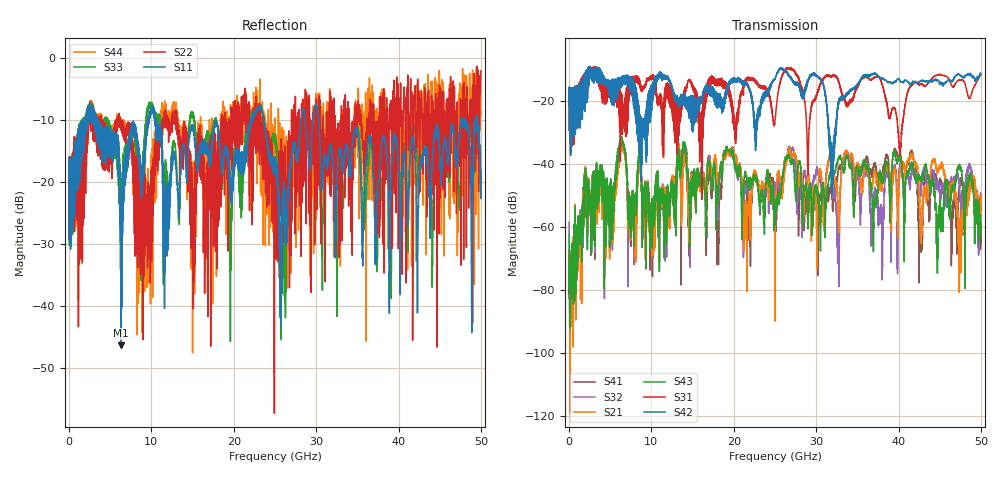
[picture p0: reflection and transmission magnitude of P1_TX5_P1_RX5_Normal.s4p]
!Keysight Technologies,N5225B,MY57041031,A.13.20.10
!Date: Friday, May 31, 2019 11:20:57
!Correction: S11(Full 4 Port(1,2,3,4))
!S12(Full 4 Port(1,2,3,4))
!S13(Full 4 Port(1,2,3,4))
!S14(Full 4 Port(1,2,3,4))
!S21(Full 4 Port(1,2,3,4))
!S22(Full 4 Port(1,2,3,4))
!S23(Full 4 Port(1,2,3,4))
!S24(Full 4 Port(1,2,3,4))
!S31(Full 4 Port(1,2,3,4))
!S32(Full 4 Port(1,2,3,4))
!S33(Full 4 Port(1,2,3,4))
!S34(Full 4 Port(1,2,3,4))
!S41(Full 4 Port(1,2,3,4))
!S42(Full 4 Port(1,2,3,4))
!S43(Full 4 Port(1,2,3,4))
!S44(Full 4 Port(1,2,3,4))
!S4P File: Measurements: <S11,S12,S13,S14>,
!<S21,S22,S23,S24>,
!<S31,S32,S33,S34>,
!<S41,S42,S43,S44>:
# Hz S  dB  R 50.0
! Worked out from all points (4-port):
!   5000 points, 10 MHz to 50 GHz, reference 50 ohm
!   strongest paths, dB at 10 MHz, 12.51 GHz, 25.01 GHz, 37.51 GHz, 50 GHz:
!     S42: -19.6, -15.7, -13.1, -12.3, -11.7
!     S31: -19.4, -23.0, -26.1, -12.3, -11.7
!     S43: -62.2, -46.0, -55.5, -47.7, -59.8
!     S21: -67.1, -44.1, -65.1, -47.2, -53.4
!     S32: -58.5, -45.8, -46.7, -55.1, -52.8
!     S41: -68.8, -44.1, -50.9, -43.8, -59.7
!   lowest |S11| = -46.4 dB at 6.34 GHz (marker M1), VSWR 1.01, Z = 49.6 - j0.26 ohm
!   |S11| at or under -10 dB: 3.502 GHz to 9.556 GHz (6.054 GHz wide, 92.7 % of centre); 10.5 GHz to 22.11 GHz (11.6 GHz wide, 71.2 % of centre); 30.29 GHz to 47.6 GHz (17.31 GHz wide, 44.4 % of centre)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
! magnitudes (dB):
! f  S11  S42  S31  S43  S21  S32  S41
! 10 MHz  -19.8  -19.6  -19.4  -62.2  -67.1  -58.5  -68.8
! 6.34 GHz  -46.4  -15.7  -20.3  -31.2  -32.9  -31.9  -32.1
! 10 GHz  -8.0  -15.8  -12.9  -54.7  -53.7  -54.6  -53.1
! 25.8 GHz  -37.9  -9.6  -12.6  -46.6  -47.7  -47.3  -45.0
! 29.88 GHz  -7.8  -11.6  -19.1  -47.8  -48.5  -44.2  -48.2
! 31.9 GHz  -15.0  -38.0  -12.2  -42.5  -39.0  -43.7  -48.6
! 50 GHz  -18.1  -11.7  -11.7  -59.8  -53.4  -52.8  -59.7
